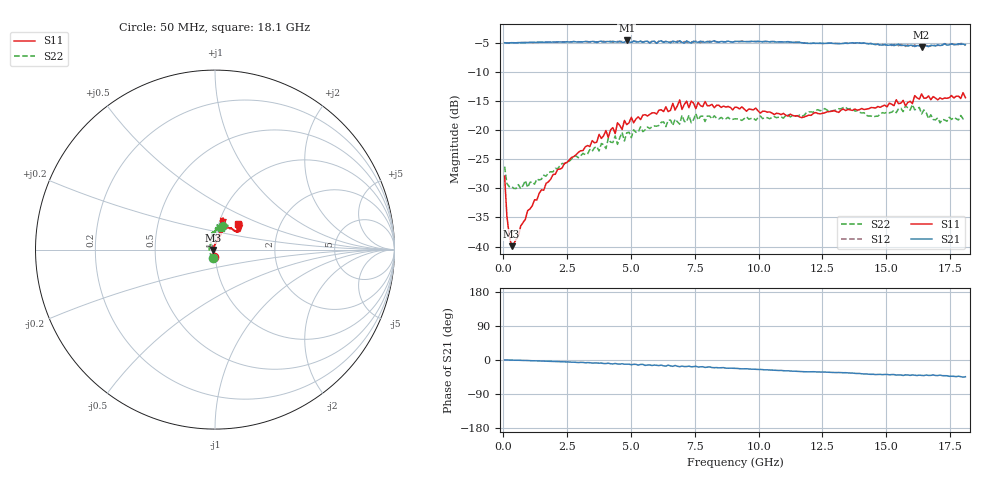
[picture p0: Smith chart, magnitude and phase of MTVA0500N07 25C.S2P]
! Network Analyzer HP8720D.06.14 Serial No. US36140669
!  5 Jul 2005  08:39:43
! Frequency  S11  S21  S12  S22
# HZ  S  DB R 50
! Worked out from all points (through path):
!   201 points, 50 MHz to 18.1 GHz, reference 50 ohm
!   highest |S21| = -4.56 dB at 4.833 GHz (marker M1); lowest = -5.7 dB at 16.39 GHz (marker M2)
!   group delay of S21, straight-line fit = 7.16 ps
!   lowest |S11| = -39.9 dB at 320.8 MHz (marker M3), VSWR 1.02, Z = 49 - j0.144 ohm
!   |S11| at or under -10 dB: start of sweep to end of sweep
!   |S22| runs from -30.1 to -15.6 dB; largest |S21 - S12| = 0.025
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5e7  -27.87 -97.8  -4.96 0.3  -4.95 0.5  -26.26 -104.8
1.4025e8  -34.84 -120.6  -5.01 0.0  -4.98 0.1  -29.15 -151.7
3.2075e8  -39.94 -171.6  -4.94 -0.2  -4.96 -0.2  -29.63 -176.7
1.6745e9  -29.14 83.7  -4.85 -3.1  -4.86 -3.1  -27.91 126.2
3.1185e9  -23.50 75.7  -4.80 -6.4  -4.83 -6.7  -23.99 109.8
4.021e9  -20.05 73.6  -4.76 -9.4  -4.82 -8.6  -23.16 100.6
4.11125e9  -21.26 73.0  -4.75 -8.4  -4.78 -9.7  -21.38 99.6
4.382e9  -20.57 71.7  -4.80 -9.1  -4.77 -10.4  -20.99 100.2
4.47225e9  -18.73 68.0  -4.83 -10.4  -4.73 -9.5  -22.43 102.9
4.83325e9  -19.04 76.7  -4.56 -10.9  -4.72 -11.7  -20.44 90.2
6.09675e9  -16.55 71.7  -4.73 -14.7  -4.65 -14.4  -19.17 87.8
6.7285e9  -16.54 77.7  -4.78 -14.4  -4.99 -15.5  -18.11 81.6
6.909e9  -14.79 75.8  -4.61 -17.7  -4.75 -16.3  -18.95 80.4
6.99925e9  -16.42 75.5  -4.89 -16.0  -4.97 -17.8  -17.42 81.7
7.17975e9  -15.02 79.9  -4.64 -17.2  -4.88 -16.4  -18.57 76.5
7.54075e9  -16.28 71.5  -4.80 -16.6  -4.66 -18.8  -17.14 85.0
9.075e9  -16.02 76.0  -4.74 -22.0  -4.72 -22.1  -18.03 74.5
1.21435e10  -17.11 62.0  -5.04 -30.9  -5.01 -31.1  -16.89 75.6
1.512175e10  -15.33 38.0  -5.36 -39.1  -5.21 -38.6  -17.00 76.6
1.602425e10  -15.43 43.5  -5.40 -39.4  -5.54 -41.5  -15.60 67.4
1.638525e10  -13.74 41.8  -5.68 -40.6  -5.48 -40.0  -17.20 63.9
1.81e10  -14.40 47.5  -5.28 -44.1  -5.44 -45.2  -17.94 74.0
